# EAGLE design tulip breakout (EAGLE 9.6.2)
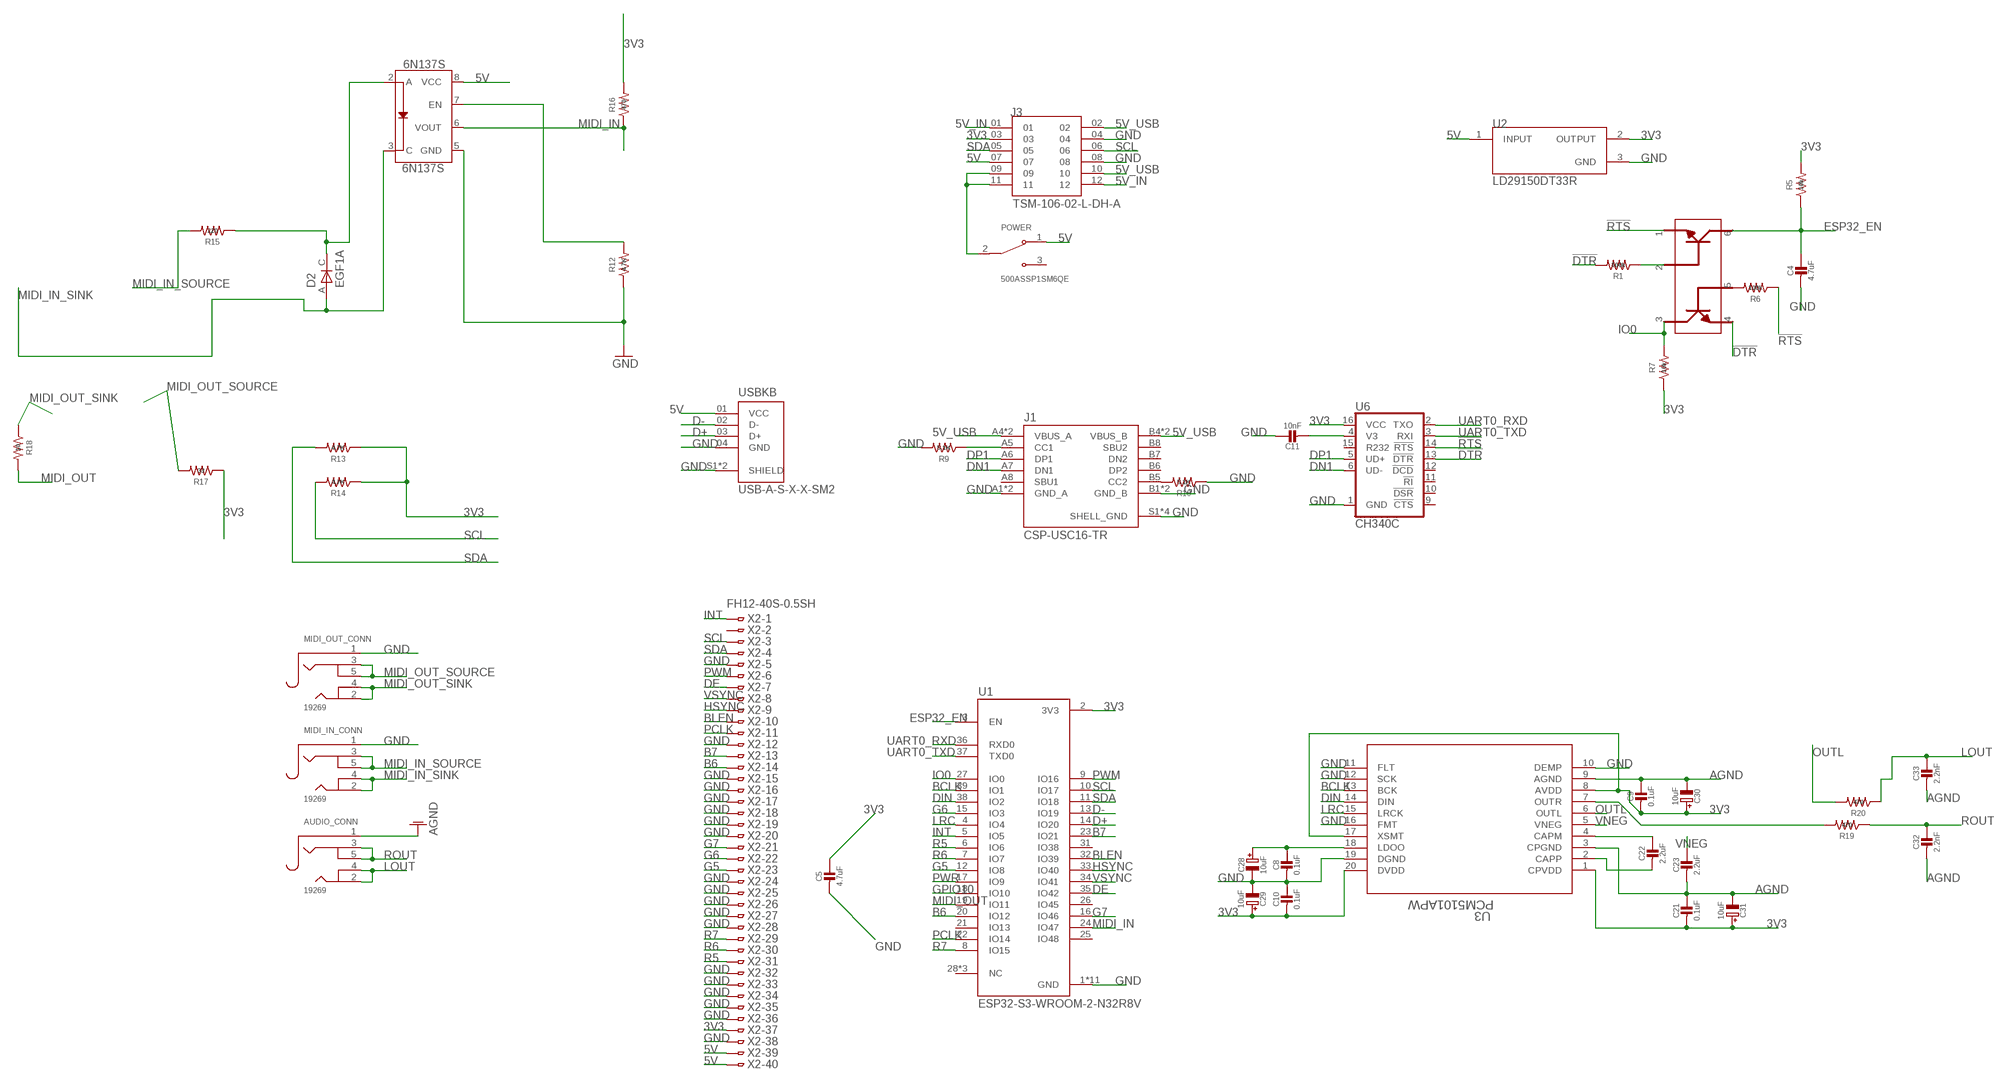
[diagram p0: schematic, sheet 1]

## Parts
6N137S  6N137S  [8-SMD]
AUDIO_CONN  19269  AUDIO_3.5MMJACK  [4UCONN_19269]
C4  4.7uF  CAP_CERAMIC0805-NOOUTLINE  [0805-NO]
C5  4.7uF  CAP_CERAMIC0805-NOOUTLINE  [0805-NO]
C8  0.1uF  CAP_CERAMIC0805-NOOUTLINE  [0805-NO]
C9  0.1uF  CAP_CERAMIC0805-NOOUTLINE  [0805-NO]
C10  0.1uF  CAP_CERAMIC0805-NOOUTLINE  [0805-NO]
C11  10nF  CAP_CERAMIC0805-NOOUTLINE  [0805-NO]
C21  0.1uF  CAP_CERAMIC0805-NOOUTLINE  [0805-NO]
C22  2.2uF  CAP_CERAMIC0805-NOOUTLINE  [0805-NO]
C23  2.2uF  CAP_CERAMIC0805-NOOUTLINE  [0805-NO]
C28  10uF  CAP_ELECTROLYTICPANASONIC_C  [PANASONIC_C]
C29  10uF  CAP_ELECTROLYTICPANASONIC_C  [PANASONIC_C]
C30  10uF  CAP_ELECTROLYTICPANASONIC_C  [PANASONIC_C]
C31  10uF  CAP_ELECTROLYTICPANASONIC_C  [PANASONIC_C]
C32  2.2nF  CAP_CERAMIC0805-NOOUTLINE  [0805-NO]
C33  2.2nF  CAP_CERAMIC0805-NOOUTLINE  [0805-NO]
D2  EGF1A  [DIOM449X264X300L114X135N]
J1  CSP-USC16-TR  [VALCON_CSP-USC16-TR]
J3  TSM-106-02-L-DH-A  [SAMTEC_TSM-106-02-L-DH-A]
MIDI_IN_CONN  19269  AUDIO_3.5MMJACK  [4UCONN_19269]
MIDI_OUT_CONN  19269  AUDIO_3.5MMJACK  [4UCONN_19269]
POWER  500ASSP1SM6QE  [SW_500ASSP1SM6QE]
R1  100k  R-US_R0805  [R0805]
R5  10k  R-US_R0805  [R0805]
R6  100k  R-US_R0805  [R0805]
R7  10k  R-US_R0805  [R0805]
R9  5.1K  R-US_R0805  [R0805]
R10  5.1K  R-US_R0805  [R0805]
R12  4.7K  R-US_R0805  [R0805]
R13  4.7K  R-US_R0805  [R0805]
R14  4.7K  R-US_R0805  [R0805]
R15  220  R-US_R0805  [R0805]
R16  470  R-US_R0805  [R0805]
R17  33  R-US_R0805  [R0805]
R18  10  R-US_R0805  [R0805]
R19  470  R-US_R0805  [R0805]
R20  470  R-US_R0805  [R0805]
RESET  MBT3904DW1T1G  [SOT236]
U1  ESP32-S3-WROOM-2-N32R8V  [XCVR_ESP32-S3-WROOM-2-N32R8V]
U2  LD29150DT33R  [DPAK456P972X240-3N]
U3  PCM5101APW  [PW20_TEX]
U6  CH340C  [SO016]
USBKB  USB-A-S-X-X-SM2  [SAMTEC_USB-A-S-X-X-SM2]
X2  FH12-40S-0.5SH  [FH12-40S-0.5SH]

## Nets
3V3: C5.1 C9.2 C10.2 C21.2 C29.+ C30.+ C31.+ J3.03 R5.2 R7.1 R13.1 R14.1 R16.2 R17.1 U1.2(3V3) U2.2(OUTPUT) U3.1(CPVDD) U3.8(AVDD) U3.17(XSMT) U3.20(DVDD) U6.16(VCC) X2.37
5V: 6N137S.8(VCC) J3.07 POWER.1(NC) U2.1(INPUT) USBKB.01(VCC) X2.39 X2.40
5V_IN: J3.01 J3.12
5V_USB: J1.A4(VBUS_A) J1.A9(VBUS_A) J1.B4(VBUS_B) J1.B9(VBUS_B) J3.02 J3.10
!DTR: R1.2 RESET.4 U6.13(!DTR)
!RTS: R6.1 RESET.1 U6.14(!RTS)
AGND: AUDIO_CONN.1 C9.1 C21.1 C23.2 C30.- C31.- C32.2 C33.2 U3.3(CPGND) U3.9(AGND)
B6: U1.20(IO12) X2.14
B7: U1.23(IO21) X2.13
BCLK: U1.39(IO1) U3.13(BCK)
BLEN: U1.32(IO39) X2.10
D+: U1.14(IO20) USBKB.03(D+)
D-: U1.13(IO19) USBKB.02(D-)
DE: U1.35(IO42) X2.7
DIN: U1.38(IO2) U3.14(DIN)
DN1: J1.A7(DN1) U6.6(UD-)
DP1: J1.A6(DP1) U6.5(UD+)
ESP32_EN: C4.1 R5.1 RESET.6 U1.3(EN)
G5: U1.12(IO8) X2.23
G6: U1.15(IO3) X2.22
G7: U1.16(IO46) X2.21
GND: 6N137S.5(GND) C4.2 C5.2 C8.2 C10.1 C11.1 C28.- C29.- J1.A1(GND_A) J1.A12(GND_A) J1.B1(GND_B) J1.B12(GND_B) J1.S1(SHELL_GND) J1.S2(SHELL_GND) J1.S3(SHELL_GND) J1.S4(SHELL_GND) J3.04 J3.08 MIDI_IN_CONN.1 MIDI_OUT_CONN.1 R9.2 R10.1 R12.1 U1.1(GND) U1.40(GND) U1.41_1(GND) U1.41_2(GND) U1.41_3(GND) U1.41_4(GND) U1.41_5(GND) U1.41_6(GND) U1.41_7(GND) U1.41_8(GND) U1.41_9(GND) U2.3(GND) U3.10(DEMP) U3.11(FLT) U3.12(SCK) U3.16(FMT) U3.19(DGND) U6.1(GND) USBKB.04(GND) USBKB.S1(SHIELD) USBKB.S2(SHIELD) X2.5 X2.12 X2.15 X2.16 X2.17 X2.18 X2.19 X2.20 X2.24 X2.25 X2.26 X2.27 X2.28 X2.32 X2.33 X2.34 X2.35 X2.36 X2.38
GPIO10: U1.18(IO10)
HSYNC: U1.33(IO40) X2.9
INT: U1.5(IO5) X2.1
IO0: R7.2 RESET.3 U1.27(IO0)
LOUT: AUDIO_CONN.2 AUDIO_CONN.4 C33.1 R20.1
LRC: U1.4(IO4) U3.15(LRCK)
MIDI_IN: 6N137S.6(VOUT) R16.1 U1.24(IO47)
MIDI_IN_SINK: 6N137S.3(C) D2.A MIDI_IN_CONN.2 MIDI_IN_CONN.4
MIDI_IN_SOURCE: MIDI_IN_CONN.3 MIDI_IN_CONN.5 R15.2
MIDI_OUT: R18.2 U1.19(IO11)
MIDI_OUT_SINK: MIDI_OUT_CONN.2 MIDI_OUT_CONN.4 R18.1
MIDI_OUT_SOURCE: MIDI_OUT_CONN.3 MIDI_OUT_CONN.5 R17.2
N$1: R1.1 RESET.2
N$2: R6.2 RESET.5
N$3: J1.B5(CC2) R10.2
N$7: C8.1 C28.+ U3.18(LDOO)
N$8: R19.2 U3.7(OUTR)
N$10: J3.09 J3.11 POWER.2(COM)
N$16: C22.1 U3.4(CAPM)
N$18: C22.2 U3.2(CAPP)
N$30: 6N137S.2(A) D2.C R15.1
N$32: 6N137S.7(EN) R12.2
N$38: C11.2 U6.4(V3)
N$42: J1.A5(CC1) R9.1
OUTL: R20.2 U3.6(OUTL)
PCLK: U1.22(IO14) X2.11
PWM: U1.9(IO16) X2.6
PWR: U1.17(IO9)
R5: U1.6(IO6) X2.31
R6: U1.7(IO7) X2.30
R7: U1.8(IO15) X2.29
ROUT: AUDIO_CONN.3 AUDIO_CONN.5 C32.1 R19.1
SCL: J3.06 R14.2 U1.10(IO17) X2.3
SDA: J3.05 R13.2 U1.11(IO18) X2.4
UART0_RXD: U1.36(RXD0) U6.2(TXO)
UART0_TXD: U1.37(TXD0) U6.3(RXI)
VNEG: C23.1 U3.5(VNEG)
VSYNC: U1.34(IO41) X2.8
Unconnected: J1.A8(SBU1) J1.B6(DP2) J1.B7(DN2) J1.B8(SBU2) POWER.3(NO) U1.21(IO13) U1.25(IO48) U1.26(IO45) U1.28(NC) U1.29(NC) U1.30(NC) U1.31(IO38) U6.9(!CTS) U6.10(!DSR) U6.11(!RI) U6.12(!DCD) U6.15(R232) X2.2

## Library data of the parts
6N137S = 6N137S:6N137S: Lite-On 6N137 - High Speed Opto Isolator Opto isolator capable of data rates up to 10MBd Check availability; AVAILABILITY: In Stock; DESCRIPTION: Logic Output Optoisolator 15MBd Open Collector 5000Vrms 1 Channel 10kV/µs CMTI 8-SMD; MF: Lite-On Inc.; MP: 6N137S; PACKAGE: SMD-8 Lite-On Inc.; PRICE: None; PURCHASE-URL: https://pricing.snapeda.com/search/part/6N137S/?ref=eda
AUDIO_CONN MIDI_IN_CONN MIDI_OUT_CONN = microbuilder:AUDIO_3.5MMJACK: 3.5MM Audio Jack These are normally connected as follows, from left-to right on the schematic symbol above: Tip: Left Audio Inner Ring: Right Audio Shell: Common/GND
C4 C5 C8-C11 C21-C23 C32 C33 = microbuilder:CAP_CERAMIC: Ceramic Capacitors
C28-C31 = microbuilder:CAP_ELECTROLYTIC: Electrolytic Capacitors
D2 = EGF1A:EGF1A: EGF1A Series 1 A 100 V 50 ns Surface Mount Fast Recovery Rectifier - DO-214AC Check availability; AVAILABILITY: In Stock; DESCRIPTION: Diode Standard 50 V 1A Surface Mount DO-214AC (SMA); MF: ON Semiconductor; MP: EGF1A; PACKAGE: SMA-2 ON Semiconductor; PRICE: None; PURCHASE-URL: https://pricing.snapeda.com/search/part/EGF1A/?ref=eda
J1 = CSP-USC16-TR:CSP-USC16-TR: CSP-USC16-TR Valcon USB Type C Surface Mount PCB Socket Check availability; AVAILABILITY: In Stock; DESCRIPTION: CSP-USC16-TR Valcon USB Type C Surface Mount PCB Socket; MF: Valcon; MP: CSP-USC16-TR; PACKAGE: None; PRICE: None; PURCHASE-URL: https://pricing.snapeda.com/search/part/CSP-USC16-TR/?ref=eda
J3 = TSM-106-02-L-DH-A:TSM-106-02-L-DH-A; DESCRIPTION: Connector Header Surface Mount, Right Angle 12 position 0.100 (2.54mm); DIGI-KEY_PART_NUMBER: 612-TSM-106-02-L-DH-A-ND; MF: Samtec; MP: TSM-106-02-L-DH-A; PACKAGE: None; PURCHASE-URL: https://pricing.snapeda.com/search/part/TSM-106-02-L-DH-A/?ref=eda
POWER = 500ASSP1SM6QE:500ASSP1SM6QE; DESCRIPTION: Slide Switch SPDT Surface Mount, Right Angle; DIGI-KEY_PART_NUMBER: EG5810TR-ND; MF: E-Switch; MP: 500ASSP1SM6QE; PACKAGE: None; PURCHASE-URL: https://pricing.snapeda.com/search/part/500ASSP1SM6QE/?ref=eda
R1 R5-R7 R9 R10 R12-R20 = adafruit:R-US_: RESISTOR, American symbol
RESET = MBT3904DW1T1G:MBT3904DW1T1G: Check availability; AVAILABILITY: In Stock; DESCRIPTION: Bipolar (BJT) Transistor Array 2 NPN (Dual) 40V 200mA 300MHz 150mW Surface Mount SC-88/SC70-6/SOT-363; MF: ON Semiconductor; MP: MBT3904DW1T1G; PACKAGE: SC-88-6 ON Semiconductor; PRICE: None; PURCHASE-URL: https://pricing.snapeda.com/search/part/MBT3904DW1T1G/?ref=eda
U1 = ESP32-S3-WROOM-2-N32R8V:ESP32-S3-WROOM-2-N32R8V: Check availability; AVAILABILITY: In Stock; DESCRIPTION: Bluetooth, WiFi 802.11b/g/n, Bluetooth v5.0 Transceiver Module 2.4GHz PCB Trace Surface Mount; MF: Espressif Systems; MP: ESP32-S3-WROOM-2-N32R8V; PACKAGE: Package; PRICE: None; PURCHASE-URL: https://pricing.snapeda.com/search/part/ESP32-S3-WROOM-2-N32R8V/?ref=eda
U2 = LD29150DT33R:LD29150DT33R: LD29150 Series 1.5 A 3.3 V Fixed Output SMT LDO Voltage Regulator - TO-252; DESCRIPTION: Linear Voltage Regulator IC Positive Fixed 1 Output 1.5A DPAK; DIGI-KEY_PART_NUMBER: 497-1496-2-ND; MF: STMicroelectronics; MP: LD29150DT33R; PACKAGE: TO-252 STMicroelectronics; PURCHASE-URL: https://pricing.snapeda.com/search/part/LD29150DT33R/?ref=eda
U3 = pcm5101apw:PCM5101APW; COPYRIGHT: Copyright (C) 2022 Ultra Librarian. All rights reserved.; DIGI-KEY_PART_NUMBER_1: PCM5101APW-ND; MANUFACTURER_PART_NUMBER: PCM5101APW; MFR_NAME: Texas Instruments
U6 = SparkFun-IC-Comms:CH340C; PROD_ID: IC-14038
USBKB = USB-A-S-X-X-SM2:USB-A-S-X-X-SM2: USB-A (USB TYPE-A) USB 2.0 Receptacle Connector 4 Position Surface Mount, Right Angle; Through Hole Check availability; AVAILABILITY: In Stock; DESCRIPTION: USB-A (USB TYPE-A) USB 2.0 Receptacle Connector 4 Position Surface Mount, Right Angle; MF: Samtec; MP: USB-A-S-F-W-SM2-TR; PACKAGE: None; PRICE: None; PURCHASE-URL: https://pricing.snapeda.com/search/part/USB-A-S-F-W-SM2-TR/?ref=eda
X2 = con-hirose:FH12-40S-0.5S: 0.5mm Pitch Connectors For FPC/FFC Source: Data sheet; MPN: FH12-40S-0.5SH(55); OC_FARNELL: 1324556; OC_NEWARK: 34M6178

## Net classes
1 power: width 0.178 mm

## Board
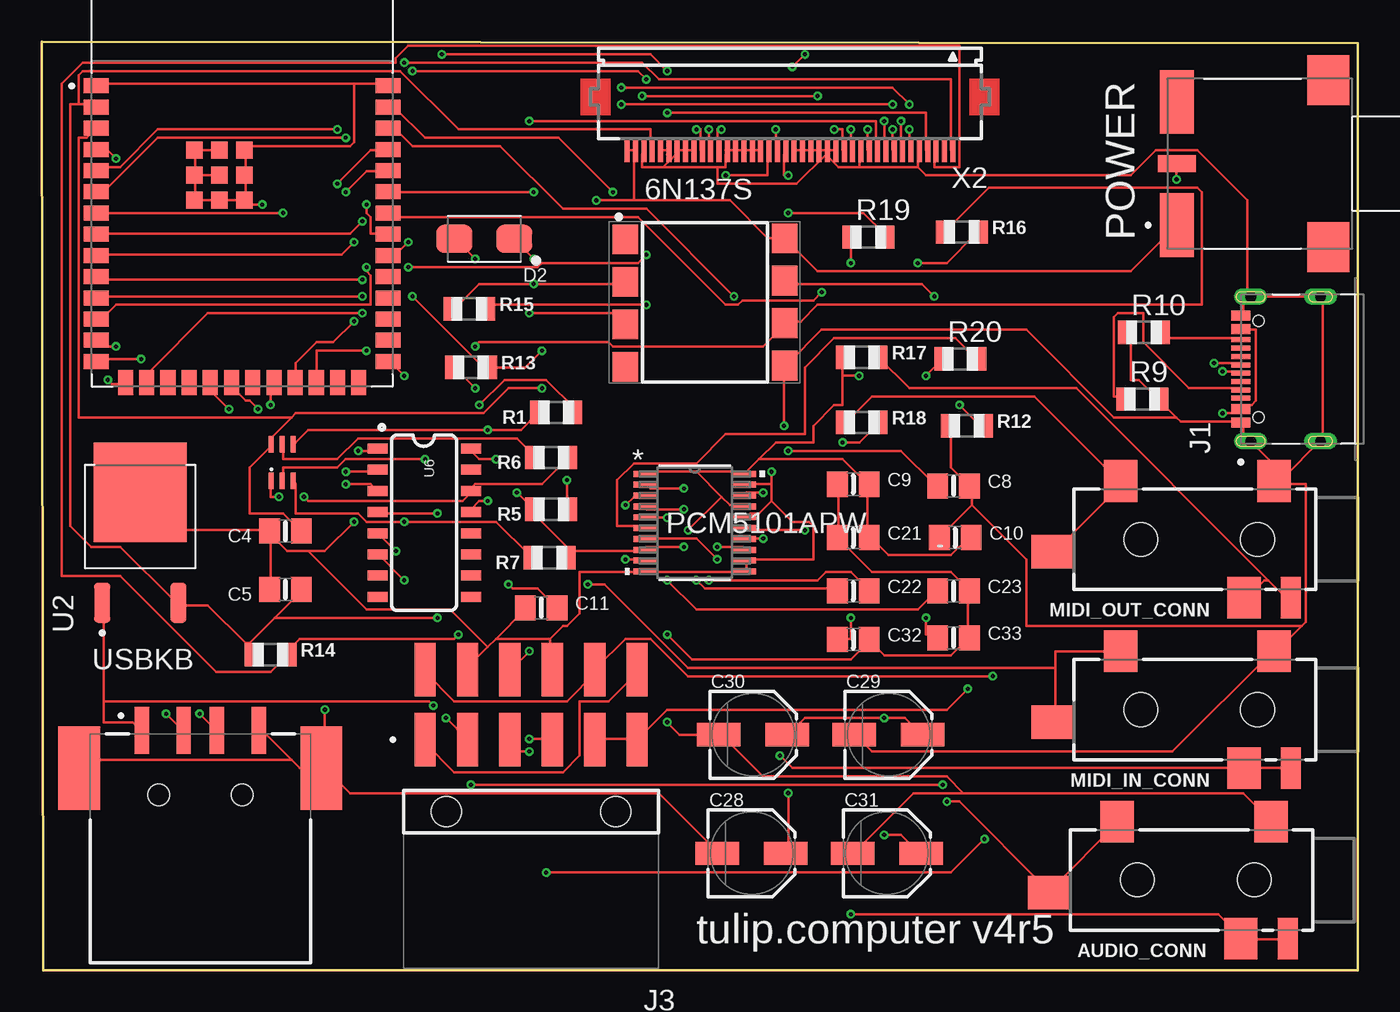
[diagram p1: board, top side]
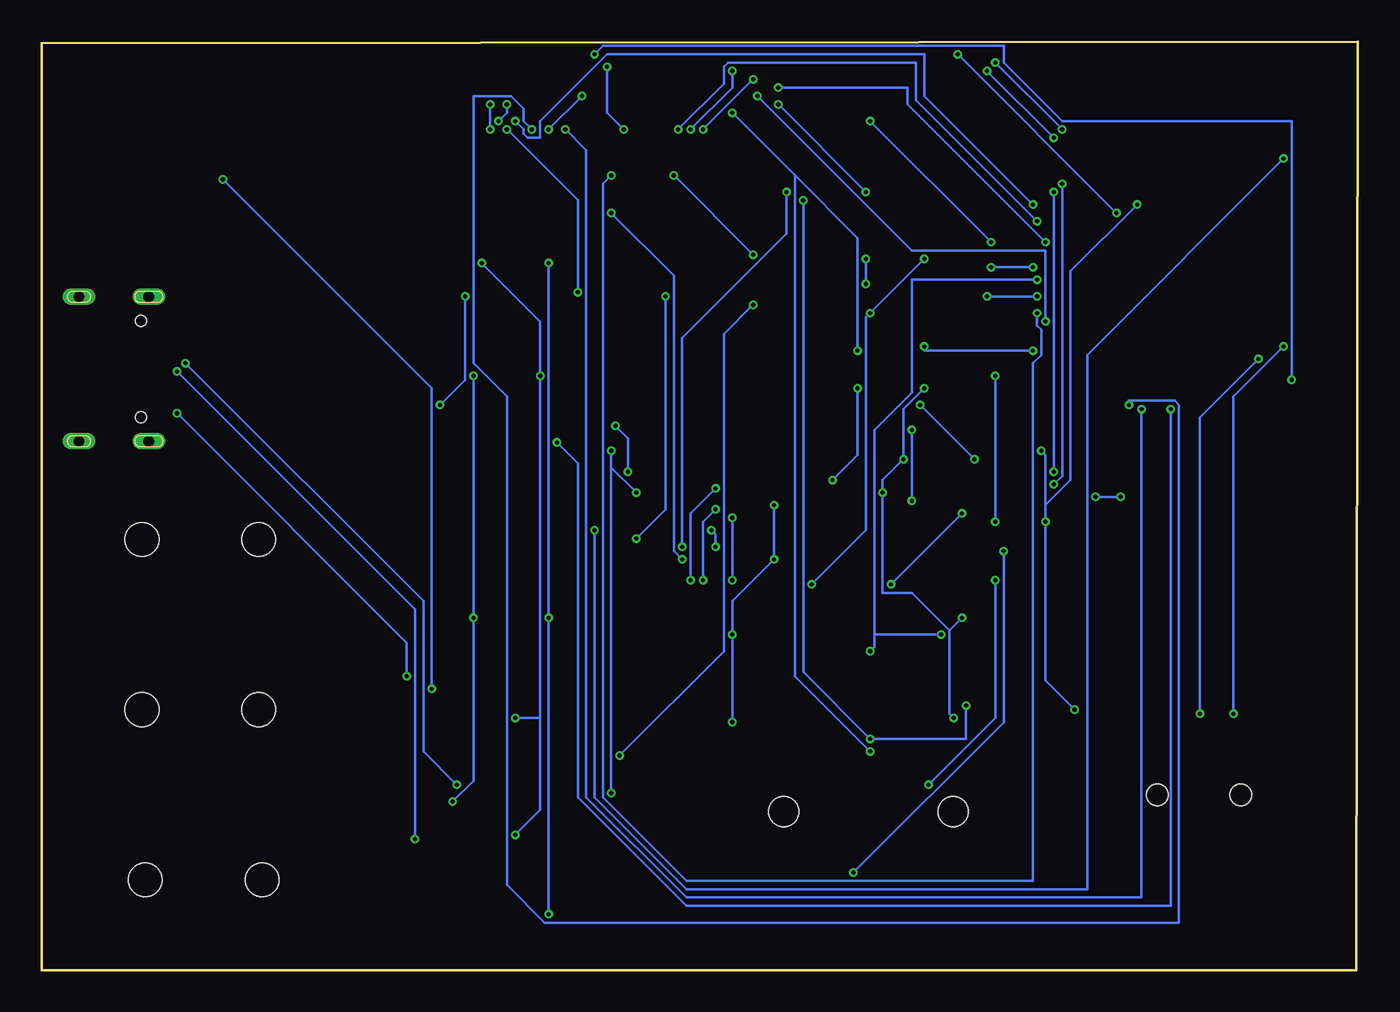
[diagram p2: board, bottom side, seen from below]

Size 78.8 x 55.6 mm. Coordinates in mm from the lower left corner, seen from the top.
Outline: 0.1,0 0,55.6 78.8,55.5 78.8,0 0.1,0
Copper layers (1*16): Top 0.035559375mm / dielectric 1.6mm / Bottom 0.035559375mm
Design rules "oshpark-2layer *": minimum track width 6mil, minimum drill 10mil, track to track 6mil, track to pad 6mil, pad to pad 6mil, via to via 6mil, smd to smd 6mil, copper to edge 0mil, drill to drill 6mil, minimum pad ring 5mil, minimum via ring 5mil, stop-mask expansion 2.5mil, vias tented up to drill 0mil, thermal gap 10mil

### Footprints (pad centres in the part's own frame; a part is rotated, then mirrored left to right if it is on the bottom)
8-SMD = smd 1.52 x 1.78: 1 -4.96,3.96; 2 -4.96,1.42; 3 -4.96,-1.12; 4 -4.96,-3.66; 5 4.58,-3.59; 6 4.58,-1.05; 7 4.58,1.49; 8 4.58,4.03
4UCONN_19269 = smd 2 x 2.5: 1 2.5,-3.5; 2 11.7,-3.5; 3 4.3,3.5 | smd 2.5 x 2: 4 15.8,0.75 | smd 1.2 x 2.5: 5 1.5,3.5 | hole 2: 3.5,0; 10.5,0
0805-NO = smd 1.24 x 1.5: 1 -0.95,0; 2 0.95,0
PANASONIC_C = smd 2.6 x 1.4: + 2.05,0; - -2.05,0
DIOM449X264X300L114X135N = smd 2.17 x 1.69: A 1.795,0; C -1.795,0
VALCON_CSP-USC16-TR = smd 0.3 x 1.14: A1 -3.35,0; A4 -2.55,0; A5 -1.25,0; A6 -0.25,0; A7 0.25,0; A8 1.25,0; A9 2.55,0; A12 3.35,0; B1 3.05,0; B4 2.25,0; B5 1.75,0; B6 0.75,0; B7 -0.75,0; B8 -1.75,0; B9 -2.25,0; B12 -3.05,0 | drill 0.65 pad 1 long: S1 -4.325,-0.59; S2 4.325,-0.59 | drill 0.65 pad 0.9 long: S3 -4.325,-4.77; S4 4.325,-4.77 | hole 0.65: -2.89,-1.07; 2.89,-1.07
SAMTEC_TSM-106-02-L-DH-A = smd 1.27 x 3.18: 01 6.35,-4.305; 02 6.35,-8.495; 03 3.81,-4.305; 04 3.81,-8.495; 05 1.27,-4.305; 06 1.27,-8.495; 07 -1.27,-4.305; 08 -1.27,-8.495; 09 -3.81,-4.305; 10 -3.81,-8.495; 11 -6.35,-4.305; 12 -6.35,-8.495 | hole 1.78: -5.08,0; 5.08,0
SW_500ASSP1SM6QE = smd 3.81 x 2.03: 1 -3.685,4.535; 3 3.685,4.535 | smd 1.02 x 2.29: 2 0,4.535 | smd 3 x 2.5: S1 -5,-4.535; S2 5,-4.535
R0805 = smd 1.1 x 1.4: 1 -1,0; 2 1,0
SOT236 = smd 0.3 x 1: 1 -0.66,-1.09; 2 0,-1.09; 3 0.66,-1.09; 4 0.66,1.09; 5 0,1.09; 6 -0.66,1.09
XCVR_ESP32-S3-WROOM-2-N32R8V = smd 1.5 x 0.9: 1 -8.75,5.26; 2 -8.75,3.99; 3 -8.75,2.72; 4 -8.75,1.45; 5 -8.75,0.18; 6 -8.75,-1.09; 7 -8.75,-2.36; 8 -8.75,-3.63; 9 -8.75,-4.9; 10 -8.75,-6.17; 11 -8.75,-7.44; 12 -8.75,-8.71; 13 -8.75,-9.98; 14 -8.75,-11.25; 27 8.75,-11.25; 28 8.75,-9.98; 29 8.75,-8.71; 30 8.75,-7.44; 31 8.75,-6.17; 32 8.75,-4.9; 33 8.75,-3.63; 34 8.75,-2.36; 35 8.75,-1.09; 36 8.75,0.18; 37 8.75,1.45; 38 8.75,2.72; 39 8.75,3.99; 40 8.75,5.26 | smd 0.9 x 1.5: 15 -6.985,-12.5; 16 -5.715,-12.5; 17 -4.445,-12.5; 18 -3.175,-12.5; 19 -1.905,-12.5; 20 -0.635,-12.5; 21 0.635,-12.5; 22 1.905,-12.5; 23 3.175,-12.5; 24 4.445,-12.5; 25 5.715,-12.5; 26 6.985,-12.5 | smd 1 x 1: 41_1 -1.36,-0.09; 41_2 -2.86,-0.09; 41_3 0.14,-0.09; 41_4 -2.86,-1.59; 41_5 -1.36,-1.59; 41_6 0.14,-1.59; 41_7 -2.86,1.41; 41_8 -1.36,1.41; 41_9 0.14,1.41
DPAK456P972X240-3N = smd 2.4 x 0.98: 1 -4.2,2.28; 2 -4.2,-2.28 | smd 5.96 x 5.57: 3 2.42,0
PW20_TEX = smd 1.473 x 0.356: 1 -2.921,2.925; 2 -2.921,2.275; 3 -2.921,1.625; 4 -2.921,0.975; 5 -2.921,0.325; 6 -2.921,-0.325; 7 -2.921,-0.975; 8 -2.921,-1.625; 9 -2.921,-2.275; 10 -2.921,-2.925; 11 2.921,-2.925; 12 2.921,-2.275; 13 2.921,-1.625; 14 2.921,-0.975; 15 2.921,-0.325; 16 2.921,0.325; 17 2.921,0.975; 18 2.921,1.625; 19 2.921,2.275; 20 2.921,2.925
SO016 = smd 0.6 x 1.2: 1 -4.445,-2.8; 2 -3.175,-2.8; 3 -1.905,-2.8; 4 -0.635,-2.8; 5 0.635,-2.8; 6 1.905,-2.8; 7 3.175,-2.8; 8 4.445,-2.8; 9 4.445,2.8; 10 3.175,2.8; 11 1.905,2.8; 12 0.635,2.8; 13 -0.635,2.8; 14 -1.905,2.8; 15 -3.175,2.8; 16 -4.445,2.8
SAMTEC_USB-A-S-X-X-SM2 = smd 0.9 x 2.8: 01 -3.5,3.85; 02 -1,3.85; 03 1,3.85; 04 3.5,3.85 | smd 2.5 x 5: S1 -7.25,1.6; S2 7.25,1.6 | hole 1.3: -2.5,0; 2.5,0
FH12-40S-0.5SH = smd 0.3 x 1.3: 1 -9.75,3.25; 2 -9.25,3.25; 3 -8.75,3.25; 4 -8.25,3.25; 5 -7.75,3.25; 6 -7.25,3.25; 7 -6.75,3.25; 8 -6.25,3.25; 9 -5.75,3.25; 10 -5.25,3.25; 11 -4.75,3.25; 12 -4.25,3.25; 13 -3.75,3.25; 14 -3.25,3.25; 15 -2.75,3.25; 16 -2.25,3.25; 17 -1.75,3.25; 18 -1.25,3.25; 19 -0.75,3.25; 20 -0.25,3.25; 21 0.25,3.25; 22 0.75,3.25; 23 1.25,3.25; 24 1.75,3.25; 25 2.25,3.25; 26 2.75,3.25; 27 3.25,3.25; 28 3.75,3.25; 29 4.25,3.25; 30 4.75,3.25; 31 5.25,3.25; 32 5.75,3.25; 33 6.25,3.25; 34 6.75,3.25; 35 7.25,3.25; 36 7.75,3.25; 37 8.25,3.25; 38 8.75,3.25; 39 9.25,3.25; 40 9.75,3.25

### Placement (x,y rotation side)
6N137S  39.9,39.8 0 top
AUDIO_CONN  76.1,5.4 180 top
C4  14.6,26.3 180 top
C5  14.6,22.8 180 top
C8  54.6,29 0 top
C9  48.6,29.1 0 top
C10  54.7,25.9 0 top
C11  29.9,21.7 0 top
C21  48.6,25.9 0 top
C22  48.6,22.7 0 top
C23  54.6,22.7 0 top
C28  42.5,7 0 top
C29  50.7,14.1 0 top
C30  42.6,14.1 0 top
C31  50.6,7 0 top
C32  48.6,19.8 0 top
C33  54.6,19.9 0 top
D2  26.5,43.8 180 top
J1  71.8,36 90 top
J3  29.3,9.5 180 top
MIDI_IN_CONN  76.3,15.6 180 top
MIDI_OUT_CONN  76.3,25.8 180 top
POWER  72.5,48.3 90 top
R1  30.8,33.4 180 top
R5  30.5,27.6 180 top
R6  30.5,30.7 180 top
R7  30.4,24.7 180 top
R9  65.9,34.2 0 top
R10  66,38.2 0 top
R12  55.4,32.6 0 top
R13  25.7,36.1 0 top
R14  13.7,18.9 0 top
R15  25.6,39.6 0 top
R16  55.1,44.2 0 top
R17  49.1,36.7 0 top
R18  49.1,32.8 0 top
R19  49.5,43.9 0 top
R20  55,36.6 0 top
RESET  14.4,30.4 0 top
U1  12,47.7 0 top
U2  5.9,26.2 90 top
U3  39.1,26.8 0 top
U6  22.9,26.8 270 top
USBKB  9.5,10.5 0 top
X2  44.8,52.3 180 top

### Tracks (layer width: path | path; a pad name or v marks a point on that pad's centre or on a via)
3V3  (via drill 0.25)
  Top 0.152: C30.+ 44.7,14.1 45.7,15.1 v50.45,15.1 51.7,15.1 52.7,14.1 C29.+ | 49.45,29.1 49.45,26.1 C21.2 49.7,25.85 50.7,24.85 54.45,24.85 55.45,25.85 C10.2 | 47.95,35.6 47.95,33.85 47.45,33.85 46.2,32.6 46.2,31.6 43.95,31.6 42.95,30.6 | 47.95,35.6 47.95,36.6 R17.1 | 42.95,30.6 42.2,29.85 U3.20 41.95,29.85 39.2,29.85 | v52.45,42.35 54.2,42.35 55.95,44.1 R16.2 | 47.95,35.6 v48.95,35.6 | 39.2,29.85 36.2,29.85 U3.1 | 39.2,29.85 40.7,28.35 | 40.7,28.35 41.2,27.85 41.95,27.85 U3.17 | v50.45,8.1 51.45,8.1 52.45,7.1 C31.+ | 49.45,29.1 47.95,30.6 42.95,30.6 | 49.45,29.1 C9.2 | 31.7,25.1 31.45,24.85 R7.1 31.7,25.1 | 31.7,25.1 35.95,25.1 U3.8 36.2,25.35 v38.45,25.35 | v27.2,30.6 26.2,30.6 25.7,31.1 U6.16 | v28.45,28.6 29.45,27.6 R5.2 29.7,27.6 29.7,27.1 31.7,25.1 | v25.95,34.85 R13.1 | v24.2,15.1 25.45,13.85 J3.03 | 12.2,19.6 9.95,21.85 8.2,21.85 U2.2 7.95,22.1 4.7,25.35 2.95,25.35 1.7,26.6 1.7,51.85 2.2,51.85 | 12.2,19.6 12.7,19.1 R14.1 | 13.95,21.1 12.45,19.6 12.2,19.6 | 13.95,21.1 15.45,22.6 C5.1 | 2.2,51.85 2.2,53.6 2.45,53.85 21.45,53.85 24.95,50.35 36.45,50.35 36.45,49.1 X2.37 | 2.2,51.85 3.2,51.85 U1.2 | 13.95,21.1 v23.7,21.1 | v38.7,26.35 40.7,28.35
  Bottom 0.152: v52.45,42.35 48.95,38.85 v48.95,35.6 48.95,15.1 | v50.45,8.1 48.95,9.6 48.95,15.1 | 48.95,15.1 v50.45,15.1 | v25.95,34.85 27.2,33.6 v27.2,30.6 28.45,29.35 v28.45,28.6 28.45,22.6 26.7,22.6 24.45,20.35 | v24.2,15.1 24.45,15.35 24.45,20.35 | v23.7,21.1 24.45,20.35 | v38.7,26.35 38.45,26.1 v38.45,25.35
5V  (via drill 0.25)
  Top 0.152: 3.7,16.1 3.7,14.85 5.45,14.85 5.95,14.35 USBKB.01 | 3.7,16.1 3.7,21.85 U2.1 | v29.2,13.85 30.45,13.85 J3.07 | v23.45,15.85 23.2,16.1 3.7,16.1 | X2.40 34.95,49.1 35.45,49.1 X2.39 35.45,48.85 35.45,46.1 | 35.45,46.1 41.2,46.1 43.45,43.85 44.45,43.85 6N137S.8 44.7,43.6 46.45,41.85 65.2,41.85 POWER.1 | 35.45,46.1 v33.2,46.1
  Bottom 0.152: v23.45,15.85 23.45,13.85 v29.2,13.85 33.2,17.85 v33.2,46.1
5V_IN
  Top 0.152: J3.01 22.95,13.6 24.7,11.85 31.2,11.85 32.2,12.85 32.2,16.1 33.95,16.1 35.7,17.85 J3.12
5V_USB  (via drill 0.25)
  Top 0.152: 71.95,33.85 71.95,33.35 J1.A4 71.7,33.35 v70.7,33.35 | 71.95,38.35 71.95,38.6 J1.A9 | 71.95,33.85 72.45,33.85 72.7,34.1 72.7,38.35 71.95,38.35 | 71.95,33.85 J1.B9 | 71.95,38.35 J1.B4 | v56.95,17.6 38.7,17.6 36.45,19.85 34.95,19.85 33.2,18.1 J3.10 33.2,17.85 31.45,16.1 24.7,16.1 22.95,17.85 J3.02
  Bottom 0.152: v70.7,33.35 56.95,19.6 v56.95,17.6
!DTR  (via drill 0.25)
  Top 0.152: RESET.4 15.2,31.6 15.95,32.35 v26.7,32.35 28.7,32.35 29.7,33.35 R1.2 | v26.7,28.1 26.2,28.1 25.7,27.6 U6.13
  Bottom 0.152: v26.7,32.35 v26.7,28.1
!RTS  (via drill 0.25)
  Top 0.152: v14.2,28.35 13.7,28.35 13.7,29.1 RESET.1 | v15.7,28.35 15.95,28.1 25.2,28.1 25.7,28.6 U6.14 25.7,28.85 25.95,29.1 29.95,29.1 31.45,30.6 R6.1
  Bottom 0.152: v15.7,28.35 v14.2,28.35
AGND  (via drill 0.25)
  Top 0.152: C9.1 47.7,29.1 47.7,26.1 C21.1 49.7,23.85 54.45,23.85 55.45,22.85 C23.2 55.45,22.6 55.45,20.1 C33.2 55.45,19.85 54.45,18.85 50.45,18.85 49.7,19.6 C32.2 49.45,19.6 48.45,18.6 38.95,18.6 v37.45,20.1 | v34.95,24.6 35.95,24.6 U3.9 | v34.95,27.85 35.45,28.35 35.95,28.35 U3.3 | 55.2,10.6 52.2,10.6 48.7,7.1 C31.- | 55.2,10.6 71.95,10.6 73.45,9.1 AUDIO_CONN.1 | 55.2,10.6 54.2,11.6 43.2,11.6 40.7,14.1 C30.- 38.2,14.1 v37.45,14.85
  Bottom 0.152: v34.95,27.85 v34.95,24.6 37.45,22.1 v37.45,20.1 v37.45,14.85
B6  (via drill 0.25)
  Top 0.152: v47.45,50.35 47.95,50.35 47.95,49.1 X2.14 | v12.95,33.6 12.45,34.1 12.2,34.1 11.2,35.1 U1.20
  Bottom 0.152: v47.45,50.35 46.2,49.1 46.2,10.35 40.2,4.35 12.95,4.35 v12.95,33.6
B7  (via drill 0.25)
  Top 0.152: v48.45,50.35 48.45,49.1 X2.13 | v35.95,52.35 v46.45,52.35 | v18.7,38.85 17.45,37.6 16.45,37.6 15.2,36.35 15.2,35.35 U1.23
  Bottom 0.152: v46.45,52.35 v48.45,50.35 | v35.95,52.35 26.7,43.1 18.7,43.1 v18.7,38.85
BCLK  (via drill 0.25)
  Top 0.152: v40.45,25.35 41.95,25.35 U3.13 | v34.2,46.6 30.95,49.85 22.95,49.85 21.2,51.6 20.95,51.6 U1.39
  Bottom 0.152: v40.45,25.35 40.45,37.85 34.2,44.1 v34.2,46.6
BLEN  (via drill 0.25)
  Top 0.152: v29.2,50.85 49.95,50.85 49.95,49.1 X2.10 | v21.95,43.6 21.2,42.85 20.95,42.85 U1.32
  Bottom 0.152: v21.95,43.6 v29.2,50.85
D+  (via drill 0.25)
  Top 0.152: v5.95,36.6 3.45,36.6 U1.14 | v9.45,15.35 10.45,14.35 USBKB.03
  Bottom 0.152: v5.95,36.6 9.45,33.1 v9.45,15.35
D-  (via drill 0.25)
  Top 0.152: v4.45,37.35 3.7,37.35 3.45,37.6 U1.13 | v7.45,15.35 8.45,14.35 USBKB.02
  Bottom 0.152: v4.45,37.35 7.45,34.35 v7.45,15.35
DE  (via drill 0.25)
  Top 0.152: v51.45,50.85 51.45,49.1 X2.7 | v34.7,51.85 v50.95,51.85 | v29.45,46.6 20.95,46.6 U1.35
  Bottom 0.152: v51.45,50.85 50.95,51.35 v50.95,51.85 | v29.45,46.6 v34.7,51.85
DIN  (via drill 0.25)
  Top 0.152: v43.2,25.85 42.2,25.85 U3.14 | v41.45,40.35 36.2,45.6 31.2,45.6 27.45,49.35 22.2,49.35 21.2,50.35 20.95,50.35 U1.38
  Bottom 0.152: v43.2,25.85 41.45,27.6 v41.45,40.35
DN1  (via drill 0.25)
  Top 0.152: v70.2,36.35 71.7,36.35 J1.A7 | v25.7,11.1 v53.95,11.1 | v21.7,23.35 20.2,24.85 U6.6
  Bottom 0.152: v70.2,36.35 55.95,22.1 55.95,13.1 v53.95,11.1 | v25.7,11.1 21.7,15.1 v21.7,23.35
DP1  (via drill 0.25)
  Top 0.152: v70.7,35.85 71.7,35.85 J1.A6 | v56.45,7.85 54.45,5.85 v30.2,5.85 | v21.2,25.1 20.2,26.1 U6.5
  Bottom 0.152: v70.7,35.85 56.45,21.6 v56.45,7.85 | v30.2,5.85 21.2,14.85 v21.2,25.1
ESP32_EN  (via drill 0.25)
  Top 0.152: C4.1 15.45,26.35 14.45,27.35 12.45,27.35 12.45,30.1 13.7,31.35 RESET.6 13.7,31.6 13.7,31.85 14.95,33.1 | v31.45,29.35 31.45,27.6 R5.1 | v29.95,34.85 27.95,34.85 26.45,33.35 15.2,33.35 14.95,33.1 | 14.95,33.1 2.2,33.1 2.2,49.85 2.7,49.85 3.2,50.35 U1.3
  Bottom 0.152: v31.45,29.35 29.95,30.85 v29.95,34.85
G5  (via drill 0.25)
  Top 0.152: v40.95,47.6 43.45,47.6 43.45,48.85 X2.23 | v36.2,42.85 35.7,42.35 29.95,42.35 29.7,42.1 v21.95,42.1 | v19.45,42.1 19.45,41.85 19.7,41.6 19.7,39.85 4.45,39.85 3.7,39.1 3.45,39.1 U1.12
  Bottom 0.152: v36.2,42.85 v40.95,47.6 | v19.45,42.1 v21.95,42.1
G6  (via drill 0.25)
  Top 0.152: v43.95,50.35 43.95,49.1 X2.22 | v45.7,54.85 v44.95,54.1 | v3.95,35.35 4.2,35.1 4.95,35.1 U1.15
  Bottom 0.152: v43.95,50.35 44.95,51.35 v44.95,54.1 | v45.7,54.85 45.2,55.35 21.2,55.35 21.2,54.35 17.7,50.85 3.95,50.85 v3.95,35.35
G7  (via drill 0.25)
  Top 0.152: v44.7,47.6 44.45,47.6 44.45,48.85 X2.21 | v19.2,39.35 9.95,39.35 6.45,35.85 6.45,35.35 U1.16
  Bottom 0.152: v44.7,47.6 45.2,47.1 45.2,10.35 40.2,5.35 19.45,5.35 19.45,36.35 18.95,36.85 18.95,38.35 19.2,38.6 v19.2,39.35
GND  (via drill 0.25)
  Top 0.152: 71.95,32.6 71.95,32.85 J1.B12 71.7,32.85 68.2,32.85 67.95,33.1 | 71.95,32.6 71.95,31.85 72.2,31.85 J1.S1 72.45,31.6 74.45,29.6 | 71.95,32.6 J1.A1 | 67.95,33.1 66.95,34.1 R9.2 66.7,34.35 65.7,35.35 65.2,35.35 65.2,38.1 R10.1 | 67.95,33.1 64.2,33.1 58.95,38.35 46.7,38.35 44.7,36.35 6N137S.5 44.45,36.1 v44.45,32.6 | 41.45,49.1 40.95,49.1 X2.28 40.95,48.85 40.95,48.1 40.45,48.1 | 41.45,49.1 41.95,49.1 | 41.45,49.1 X2.27 | 41.95,49.1 42.45,49.1 | 41.95,49.1 X2.26 | 42.45,49.1 42.95,49.1 X2.24 | 42.45,49.1 X2.25 | X2.36 36.95,49.1 37.45,49.1 X2.35 37.45,48.85 37.7,48.6 | 37.2,48.1 35.95,48.1 35.95,48.85 X2.38 | 37.7,48.6 37.95,48.85 X2.34 37.95,49.1 38.45,49.1 | 37.7,48.6 37.2,48.1 | 38.45,49.1 38.95,49.1 X2.32 | 38.45,49.1 X2.33 | 37.2,48.1 40.45,48.1 | 45.45,49.1 44.95,49.1 X2.20 | 45.45,49.1 45.95,49.1 | 45.45,49.1 X2.19 | 45.95,49.1 46.45,49.1 | 45.95,49.1 X2.18 | 46.45,49.1 46.95,49.1 | 46.45,49.1 X2.17 | 46.95,49.1 47.45,49.1 X2.15 | 46.95,49.1 X2.16 46.95,48.85 | 48.95,48.1 48.95,48.85 X2.12 | 48.95,48.1 47.7,48.1 46.95,48.85 | 52.45,48.1 52.45,48.85 X2.5 | 48.95,48.1 52.45,48.1 | 40.45,48.1 40.45,47.1 45.2,47.1 46.95,48.85 | R12.1 54.45,32.6 54.45,30.1 C8.2 55.7,28.85 55.7,27.85 | 55.7,27.85 C10.1 | 71.95,39.35 71.95,39.1 J1.B1 | 71.95,39.35 71.95,40.1 72.2,40.1 J1.S2 | 71.95,39.35 J1.A12 | J1.S2 72.45,40.35 76.45,40.35 J1.S4 76.7,40.1 76.7,31.85 J1.S3 76.45,31.6 74.45,29.6 | 74.45,29.6 74.2,29.35 73.95,29.35 MIDI_OUT_CONN.1 | 75.45,20.6 75.7,20.85 75.7,29.1 73.95,29.1 MIDI_OUT_CONN.1 | 75.45,20.6 73.95,19.1 MIDI_IN_CONN.1 73.7,19.1 67.7,13.1 49.7,13.1 48.7,14.1 C29.- | 55.7,27.85 58.95,24.6 58.95,20.6 75.45,20.6
  Top 0.152: 52.45,48.1 52.95,47.6 65.2,47.6 66.7,49.1 69.2,49.1 72.2,46.1 72.2,40.35 J1.S2 | 74.45,29.6 MIDI_OUT_CONN.1 | 16.95,12.1 18.45,10.6 36.95,10.6 40.45,7.1 C28.- | 14.95,12.6 15.45,12.1 USBKB.S2 16.95,12.1 | 14.95,12.6 13.2,14.35 USBKB.04 | 14.95,12.6 2.95,12.6 2.45,12.1 USBKB.S1 | 26.7,19.35 25.45,18.1 J3.04 | 26.7,19.35 27.2,19.85 | 27.2,19.85 28.95,21.6 C11.1 | 30.45,19.85 30.45,18.1 J3.08 | 27.2,19.85 30.45,19.85 | 43.7,28.1 42.95,27.35 42.45,27.35 42.2,27.1 U3.16 | 43.7,29.1 43.7,28.1 | 43.7,29.1 42.2,29.1 U3.19 | 43.7,28.1 44.95,26.85 45.95,26.85 46.2,26.6 46.2,24.6 42.2,24.6 U3.12 42.2,24.35 42.2,23.85 U3.11 41.95,23.85 36.2,23.85 U3.10 35.95,23.85 32.2,23.85 32.2,21.35 31.45,20.6 31.2,20.6 30.45,19.85 | 9.2,49.1 10.45,49.1 U1.41_8 | 9.2,47.6 10.45,47.6 U1.41_1 | U1.41_6 11.95,46.1 10.7,46.1 U1.41_5 10.45,46.1 9.2,46.1 U1.41_4 9.2,46.35 9.2,47.6 | U1.41_6 12.2,46.35 12.2,47.6 U1.41_3 12.2,47.85 12.2,49.1 U1.41_9 12.2,49.35 18.45,49.35 18.7,49.6 18.7,53.1 | 9.2,47.6 U1.41_2 9.2,47.85 9.2,49.1 | 9.2,49.1 U1.41_7 | 18.7,53.1 20.7,53.1 U1.40 | 18.7,53.1 3.45,53.1 U1.1 | v18.95,31.1 19.95,31.1 U6.1 | v18.7,26.85 16.95,25.1 15.95,25.1 | 15.95,25.1 14.7,25.1 13.7,26.1 | 13.7,26.1 13.7,22.85 C5.2 | 13.7,26.1 C4.2 13.45,26.35 8.2,26.35 5.95,28.6 U2.3 | v13.2,45.85 12.45,45.85 12.2,46.1 U1.41_6 | 26.7,19.35 24.45,21.6 19.45,21.6 15.95,25.1 | v16.95,15.6 16.95,12.1 | 43.7,29.1 v43.7,29.85
  Bottom 0.152: v18.95,31.1 18.7,30.85 18.7,27.85 | 18.7,27.85 v18.7,26.85 18.7,17.35 v16.95,15.6 | v13.2,45.85 17.2,41.85 17.2,29.35 18.7,27.85 | v44.45,32.6 43.7,31.85 v43.7,29.85
HSYNC  (via drill 0.25)
  Top 0.152: v50.45,50.85 50.45,49.1 X2.9 | v19.45,45.85 19.45,45.35 19.7,45.1 19.7,44.1 20.7,44.1 U1.33
  Bottom 0.152: v50.45,50.85 49.95,50.35 49.95,50.1 49.7,49.85 48.95,49.85 48.95,50.85 44.95,54.85 25.95,54.85 25.95,52.35 v19.45,45.85
INT  (via drill 0.25)
  Top 0.152: v21.7,54.35 35.95,54.35 36.95,53.35 54.45,53.35 54.45,49.1 X2.1 | v17.7,50.35 6.95,50.35 4.7,48.1 3.45,48.1 U1.5
  Bottom 0.152: v17.7,50.35 v21.7,54.35
IO0  (via drill 0.25)
  Top 0.152: RESET.3 15.2,29.1 15.2,27.35 18.95,27.35 19.45,26.85 v21.7,26.85 27.2,26.85 29.2,24.85 R7.2 | v21.7,35.6 20.95,36.35 U1.27
  Bottom 0.152: v21.7,26.85 v21.7,35.6
LOUT  (via drill 0.25)
  Top 0.152: AUDIO_CONN.2 64.45,8.85 60.45,4.85 AUDIO_CONN.4 60.2,4.85 54.95,10.1 v54.2,10.1 | v52.95,35.6 53.95,36.6 R20.1 | v52.95,21.1 52.95,20.1 53.45,20.1 C33.1
  Bottom 0.152: v52.95,35.6 v52.95,21.1 52.95,11.35 v54.2,10.1
LRC  (via drill 0.25)
  Top 0.152: v45.7,26.35 42.2,26.35 U3.15 | v4.45,48.6 3.95,49.1 3.45,49.1 U1.4
  Bottom 0.152: v45.7,26.35 45.7,10.35 40.2,4.85 16.2,4.85 16.2,36.85 v4.45,48.6
MIDI_IN  (via drill 0.25)
  Top 0.152: R16.1 54.2,44.35 56.7,46.85 69.2,46.85 69.45,46.6 69.45,39.85 46.45,39.85 45.45,38.85 44.7,38.85 6N137S.6 44.45,38.6 43.2,37.35 34.2,37.35 33.95,37.6 26.2,37.6 v25.95,37.35 | v19.45,37.1 16.45,37.1 16.45,35.35 U1.24
  Bottom 0.152: v19.45,37.1 25.95,37.1 v25.95,37.35
MIDI_IN_SINK  (via drill 0.25)
  Top 0.152: 60.7,18.1 60.7,19.1 MIDI_IN_CONN.2 | 60.7,18.1 60.7,14.85 MIDI_IN_CONN.4 | v29.2,39.35 34.2,39.35 34.7,38.85 6N137S.3 | v25.95,42.6 24.95,43.6 D2.A | 60.7,18.1 38.7,18.1 33.7,23.1 v32.7,23.1
  Bottom 0.152: v25.95,42.6 v29.2,39.35 29.45,39.1 29.45,26.35 v32.7,23.1
MIDI_IN_SOURCE  (via drill 0.25)
  Top 0.152: v36.2,39.85 26.95,39.85 26.7,39.6 R15.2 | v44.2,12.85 44.95,12.1 MIDI_IN_CONN.3 MIDI_IN_CONN.5
  Bottom 0.152: v36.2,39.85 37.95,38.1 37.95,19.1 v44.2,12.85
MIDI_OUT  (via drill 0.25)
  Top 0.152: v47.95,31.6 48.95,31.6 49.95,32.6 R18.2 | v11.2,33.6 10.2,34.6 10.2,35.1 U1.19
  Bottom 0.152: v47.95,31.6 46.7,30.35 46.7,10.35 40.2,3.85 11.2,3.85 v11.2,33.6
MIDI_OUT_SINK
  Top 0.152: R18.1 48.2,32.85 49.7,34.35 59.45,34.35 64.45,29.35 MIDI_OUT_CONN.2 64.7,29.1 60.7,25.1 MIDI_OUT_CONN.4
MIDI_OUT_SOURCE
  Top 0.152: R17.2 51.95,34.85 61.95,34.85 73.45,23.35 | 73.45,23.35 74.45,22.35 74.7,22.35 MIDI_OUT_CONN.5 | 73.45,23.35 73.2,23.35 72.2,22.35 MIDI_OUT_CONN.3
N$1  (via drill 0.25)
  Top 0.152: v22.95,30.6 18.2,30.6 17.7,30.1 14.45,30.1 14.45,29.35 RESET.2 | v26.2,33.85 27.7,35.35 30.2,35.35 31.95,33.6 R1.1
  Bottom 0.152: v26.2,33.85 v22.95,30.6
N$2
  Top 0.152: RESET.5 14.45,31.35 14.45,30.6 17.7,30.6 18.95,31.85 28.45,31.85 29.45,30.85 R6.2
N$3
  Top 0.152: J1.B5 71.7,37.85 67.45,37.85 67.2,38.1 R10.2
N$7  (via drill 0.25)
  Top 0.152: v43.2,28.6 42.2,28.6 U3.18 | v44.7,31.1 51.45,31.1 53.45,29.1 C8.1 | v44.7,10.6 44.7,7.1 C28.+
  Bottom 0.152: 44.7,30.1 v43.2,28.6 | v44.7,31.1 44.7,30.1 | 44.7,30.1 v44.7,10.6
N$8  (via drill 0.25)
  Top 0.152: v44.7,45.35 49.2,45.35 50.45,44.1 R19.2 | v40.45,24.6 39.2,25.85 36.2,25.85 U3.7
  Bottom 0.152: v44.7,45.35 40.95,41.6 40.95,25.1 v40.45,24.6
N$10  (via drill 0.25)
  Top 0.152: v67.95,47.35 67.95,48.1 POWER.2 | v55.45,16.85 54.2,15.6 37.45,15.6 35.7,13.85 J3.11 35.45,13.85 33.2,13.85 J3.09
  Bottom 0.152: v67.95,47.35 55.45,34.85 v55.45,16.85
N$16  (via drill 0.25)
  Top 0.152: v38.45,27.6 36.2,27.6 U3.4 | v39.2,23.35 39.7,22.85 47.45,22.85 C22.1
  Bottom 0.152: v38.45,27.6 39.2,26.85 v39.2,23.35
N$18  (via drill 0.25)
  Top 0.152: v38.45,28.85 36.45,28.85 36.2,29.1 U3.2 | v39.95,23.35 46.45,23.35 46.95,23.85 48.45,23.85 49.45,22.85 C22.2
  Bottom 0.152: v38.45,28.85 39.95,27.35 v39.95,23.35
N$30  (via drill 0.25)
  Top 0.152: R15.1 24.7,39.6 26.2,41.1 v29.45,41.1 34.7,41.1 6N137S.2 | v29.45,42.6 28.45,43.6 D2.C
  Bottom 0.152: v29.45,41.1 v29.45,42.6
N$32  (via drill 0.25)
  Top 0.152: v54.95,33.85 56.2,32.6 R12.2 | v53.45,40.35 52.7,41.1 44.7,41.1 6N137S.7
  Bottom 0.152: v54.95,33.85 53.45,35.35 v53.45,40.35
N$38  (via drill 0.25)
  Top 0.152: v23.7,27.35 20.2,27.35 U6.4 | v27.95,23.1 28.2,22.85 29.7,22.85 C11.2
  Bottom 0.152: v27.95,23.1 v23.7,27.35
N$42
  Top 0.152: J1.A5 71.7,34.85 68.7,34.85 65.95,37.6 65.95,39.35 64.45,39.35 64.2,39.1 64.2,34.35 64.7,34.35 R9.1
OUTL
  Top 0.152: R20.2 55.95,36.6 54.7,37.85 47.45,37.85 45.7,36.1 45.7,32.1 40.95,32.1 39.2,30.35 35.45,30.35 34.45,29.35 34.45,26.6 35.95,26.6 U3.6
PCLK  (via drill 0.25)
  Top 0.152: v49.45,50.35 49.45,49.1 X2.11 | v13.7,33.85 13.7,35.1 U1.22
  Bottom 0.152: v49.45,50.35 49.95,50.85 49.95,51.6 50.7,52.35 52.95,52.35 52.95,36.35 50.95,34.35 50.95,5.1 48.7,2.85 10.7,2.85 10.7,33.85 10.95,34.1 13.7,34.1 v13.7,33.85
PWM  (via drill 0.25)
  Top 0.152: v51.95,50.35 51.95,49.1 X2.6 | v51.95,51.85 50.95,52.85 v34.7,52.85 | v18.7,43.6 17.95,42.85 3.45,42.85 U1.9
  Bottom 0.152: v51.95,51.85 v51.95,50.35 | v34.7,52.85 26.95,52.85 26.95,51.85 v18.7,43.6
R5  (via drill 0.25)
  Top 0.152: v39.2,50.35 39.45,50.35 39.45,49.1 X2.31 | v36.2,53.35 35.7,53.85 v22.2,53.85 | v18.2,49.85 6.95,49.85 3.95,46.85 3.45,46.85 U1.6
  Bottom 0.152: v36.2,53.35 v39.2,50.35 | v18.2,49.85 v22.2,53.85
R6  (via drill 0.25)
  Top 0.152: v39.95,50.35 39.95,49.1 X2.30 | v37.45,53.85 36.45,54.85 v23.95,54.85 | v14.45,45.35 3.45,45.35 U1.7
  Bottom 0.152: v39.95,50.35 37.45,52.85 v37.45,53.85 | v14.45,45.35 v23.95,54.85
R7  (via drill 0.25)
  Top 0.152: v40.7,50.35 40.45,50.35 40.45,49.1 X2.29 | v19.2,44.85 18.45,44.1 3.45,44.1 U1.8
  Bottom 0.152: v40.7,50.35 37.95,53.1 37.95,54.1 37.7,54.35 26.45,54.35 26.45,52.1 v19.2,44.85
ROUT  (via drill 0.25)
  Top 0.152: AUDIO_CONN.5 74.45,1.85 71.95,1.85 AUDIO_CONN.3 71.7,2.1 70.45,3.35 v48.45,3.35 | v48.45,42.35 48.45,43.85 R19.1 | v48.45,21.1 48.45,19.85 47.7,19.85 C32.1
  Bottom 0.152: v48.45,42.35 v48.45,21.1 v48.45,3.35
SCL  (via drill 0.25)
  Top 0.152: v19.2,41.35 3.45,41.35 U1.10 | v29.2,19.1 28.2,18.1 J3.06 | X2.3 53.45,48.85 53.45,48.1 54.95,48.1 54.95,55.35 21.95,55.35 21.2,54.6 21.2,54.35 2.45,54.35 1.2,53.1 1.2,23.6 4.7,23.6 10.45,17.85 13.7,17.85 14.7,18.85 R14.2 14.7,19.1 15.45,19.85 24.7,19.85 v24.95,20.1
  Bottom 0.152: v19.2,41.35 26.7,41.35 26.7,34.6 28.95,32.35 28.95,20.1 | 28.95,20.1 28.95,19.35 v29.2,19.1 | v24.95,20.1 28.95,20.1
SDA  (via drill 0.25)
  Top 0.152: v37.45,51.35 52.95,51.35 52.95,49.1 X2.4 | v29.95,37.1 28.95,36.1 R13.2 26.45,36.1 v22.2,40.35 | v19.2,40.35 3.45,40.35 U1.11 | v29.2,13.1 28.7,13.1 28.2,13.6 J3.05
  Bottom 0.152: 33.7,47.6 29.95,43.85 v29.95,37.1 | 33.7,47.6 v37.45,51.35 | v22.2,40.35 v19.2,40.35 | v29.2,13.1 33.7,17.6 33.7,47.6
UART0_RXD  (via drill 0.25)
  Top 0.152: v18.2,29.85 19.95,29.85 U6.2 | v18.2,46.6 19.45,47.85 20.7,47.85 U1.36
  Bottom 0.152: v18.2,46.6 v18.2,29.85
UART0_TXD  (via drill 0.25)
  Top 0.152: v18.2,29.1 19.7,29.1 19.95,28.85 U6.3 | v17.7,47.1 19.7,49.1 20.7,49.1 U1.37
  Bottom 0.152: v18.2,29.1 17.7,29.6 v17.7,47.1
VNEG  (via drill 0.25)
  Top 0.152: v37.45,27.1 36.2,27.1 U3.5 | v37.45,23.35 39.2,21.6 52.45,21.6 53.45,22.6 C23.1
  Bottom 0.152: v37.45,23.35 v37.45,27.1
VSYNC  (via drill 0.25)
  Top 0.152: v50.95,50.35 50.95,49.1 X2.8 | v46.7,40.6 46.2,40.1 41.95,40.1 41.7,39.85 40.95,39.85 35.7,45.1 20.95,45.1 U1.34
  Bottom 0.152: v50.95,50.35 46.7,46.1 v46.7,40.6

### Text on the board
tNames: tulip.computer v4r5
tValues: Close
Measures: All dimensions in inches | Units: Inches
